(* Logix 5000 AddOnInstructionDefinition export AKD_Get_Parameter_LINT; software revision 19.01 *)

TYPE AKD_Status :   // All connections to the drive ethernet module are established and data is successfully transferring.
STRUCT
   Profile_In_Progress : BOOL;   // Profile Move In Progress
   Block_In_Execution : BOOL;   // Block In Execution
   On_Target_Position : BOOL;   // On Target Position (1=Current Position Equals Last Target Position)
   General_Fault : BOOL;   // General Fault
   Current_Direction : BOOL;   // Current Motor Direction (0=Reverse, 1=Forward)
   Home_Level : BOOL;   // Level of Home Input
   Reg_Level : BOOL;   // Level of Registration Input
   Enable : BOOL;   // State of Enable Output
   Fault_Input_Fault : BOOL;   // Fault Input Active
   Fwd_Limit : BOOL;   // Forward Input Active
   Rev_Limit : BOOL;   // Reverse Input Active
   Positive_Limit : BOOL;   // Positive Software Limit Exceeded
   Negative_Limit : BOOL;   // Negative Software Limit Exceeded
   FE_Fault : BOOL;   // Following Error Fault
   Block_Fault : BOOL;   // Block Execution Fault
   Load_Complete : BOOL;   // Command Message Successfully Loaded
END_STRUCT
END_TYPE

TYPE AKD_Control :   // Send Explicit Message
STRUCT
   Load_Data_Start_Profile : BOOL;   // Load Command Data / Start Profile Move
   Start_Block : BOOL;   // Execute Command block or block chain
   Incremental : BOOL;   // Incremental Position (0=Absolute, 1=Incremental)
   Direction : BOOL;   // Direction in Velocity Mode (0=Reverse, 1=Forward)
   Smooth_Stop : BOOL;   // Smooth / Controlled Stop w/ Deceleration
   Hard_Stop : BOOL;   // Hard / Immediate Stop
   Reg_Arm : BOOL;   // Arm the Registration Input
   Enable : BOOL;   // Enable Output
END_STRUCT
END_TYPE

TYPE AKD_Axis :   // Axis Data:
STRUCT
   Control : AKD_Control;   // Control bits to send to the drive
   Status : AKD_Status;   // Status bits received from the drive
   Input : AB:ETHERNET_MODULE_SINT_64Bytes:I:0;   // Data from the drive
   Output : AB:ETHERNET_MODULE_SINT_64Bytes:O:0;   // Data to the drive
   ResponseMsgType : SINT;   // Response type contained in latest IO response from drive. Used to check for errors
   CommandTimeout : INT;   // Time to allow for command response from drive. Dependent on scan rate and communicaiton rate
   PositionFeedback : DINT;   // Actual Position Value
   VelocityFeedback : DINT;   // Actual Velocity Value
END_STRUCT
END_TYPE

ADD_ON_INSTRUCTION AKD_Get_Parameter_LINT   (* revision 0.0, ExecutePrescan, ExecuteEnableInFalse *)
// Get 8 byte Drive Parameter
VAR_OUTPUT
   DN : BOOL; {access Read Only, visible}   // Command Successful
   ER : BOOL; {access Read Only, visible}   // Error
END_VAR
VAR_IN_OUT
   Axis : AKD_Axis; {required}
END_VAR
VAR_INPUT
   Parameter_Number : INT; {visible}   // See help (F1) for parameter list.
END_VAR
VAR_OUTPUT
   Parameter_Value_LSB : DINT; {access Read Only, required}   // Lower Parameter Value
   Parameter_Value_MSB : DINT; {access Read Only, required}   // Upper Parameter Value
END_VAR
VAR
   Command_Timeout : TIMER := (PRE := 2000);   // Timeout Timer
   Command_Message_Type : SINT;   // Command Message Type
   Command_Axis_Number : SINT;   // Command Axis Number
   Step : SINT;
   Command_Bytes : SINT[8];
   OS_LoadStart : BOOL;
   Temp_Bytes : SINT[2];   // Temporary Bytes to Split into Command Bytes
END_VAR

ROUTINE EnableInFalse   (* ladder *)
// EnableIn_False
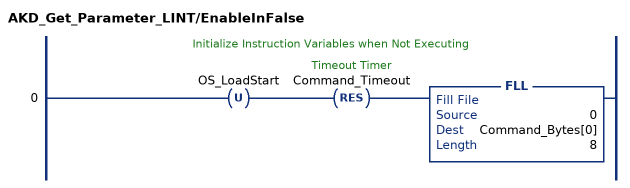
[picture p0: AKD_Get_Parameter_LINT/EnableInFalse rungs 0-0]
   // Initialize Instruction Variables when Not Executing
   0: OTU(OS_LoadStart)RES(Command_Timeout)FLL(0,Command_Bytes[0],8);
END_ROUTINE

ROUTINE Logic   (* ladder *)
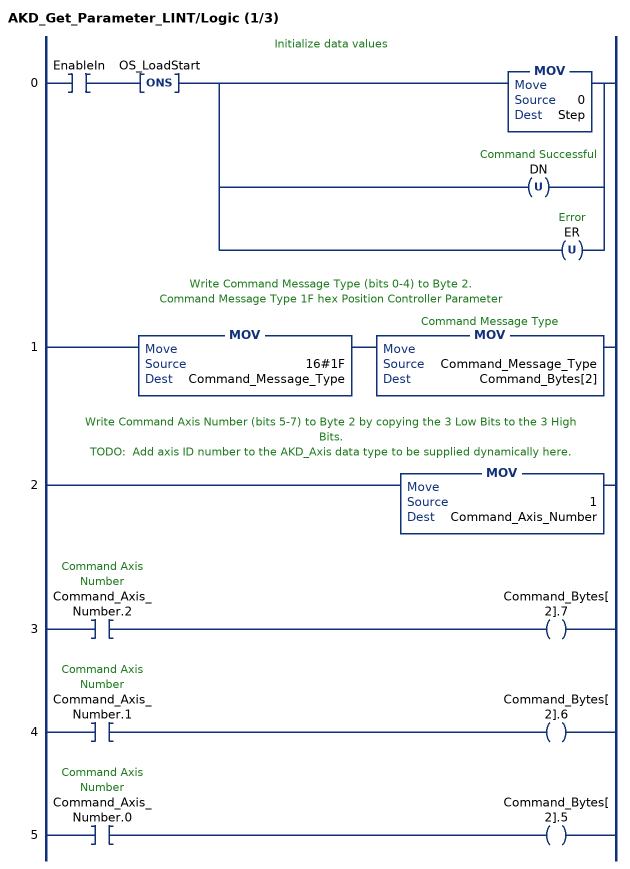
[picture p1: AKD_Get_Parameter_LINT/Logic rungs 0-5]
   // Initialize data values
   0: XIC(EnableIn)ONS(OS_LoadStart)[MOV(0,Step) ,OTU(DN) ,OTU(ER) ];
   // Write Command Message Type (bits 0-4) to Byte 2.
   // Command Message Type 1F hex Position Controller Parameter
   1: MOV(16#1F,Command_Message_Type)MOV(Command_Message_Type,Command_Bytes[2]);
   // Write Command Axis Number (bits 5-7) to Byte 2 by copying the 3 Low Bits to the 3 High Bits.
   // TODO:  Add axis ID number to the AKD_Axis data type to be supplied dynamically here.
   2: MOV(1,Command_Axis_Number);
   3: XIC(Command_Axis_Number.2)OTE(Command_Bytes[2].7);
   4: XIC(Command_Axis_Number.1)OTE(Command_Bytes[2].6);
   5: XIC(Command_Axis_Number.0)OTE(Command_Bytes[2].5);
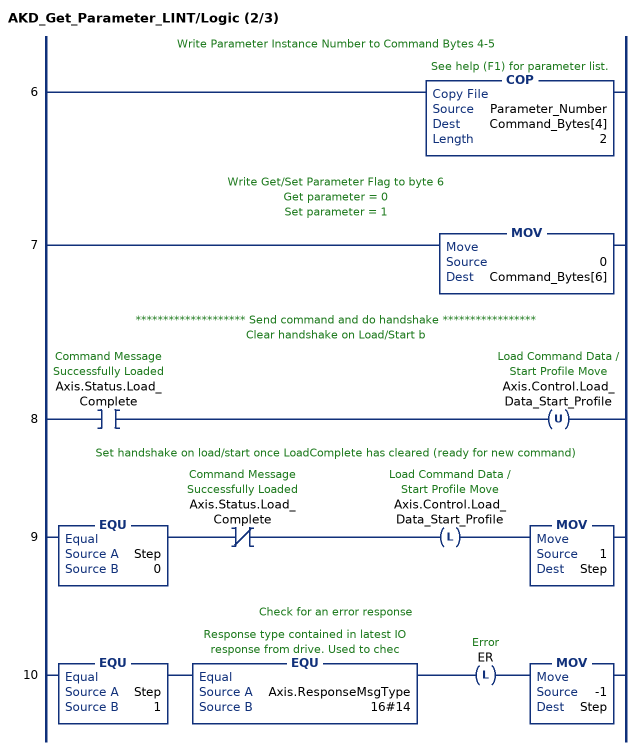
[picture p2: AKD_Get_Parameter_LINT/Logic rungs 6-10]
   // Write Parameter Instance Number to Command Bytes 4-5
   6: COP(Parameter_Number,Command_Bytes[4],2);
   // Write Get/Set Parameter Flag to byte 6
   // Get parameter = 0
   // Set parameter = 1
   7: MOV(0,Command_Bytes[6]);
   // ******************** Send command and do handshake *****************
   // Clear handshake on Load/Start b
   8: XIC(Axis.Status.Load_Complete)OTU(Axis.Control.Load_Data_Start_Profile);
   // Set handshake on load/start once LoadComplete has cleared (ready for new command)
   9: EQU(Step,0)XIO(Axis.Status.Load_Complete)OTL(Axis.Control.Load_Data_Start_Profile)MOV(1,Step);
   // Check for an error response
   10: EQU(Step,1)EQU(Axis.ResponseMsgType,16#14)OTL(ER)MOV(-1,Step);
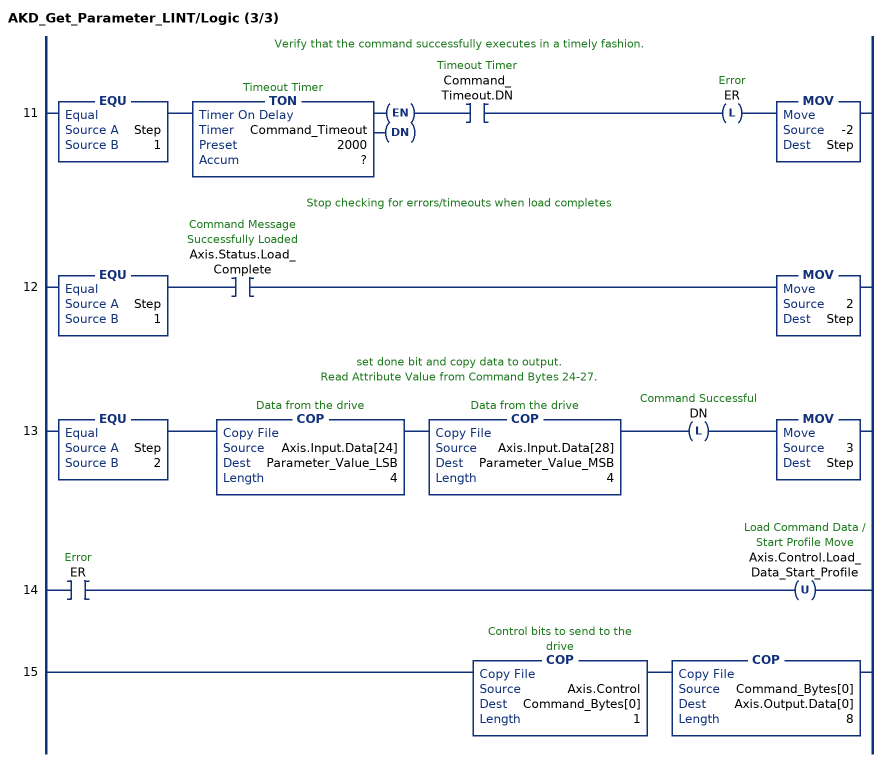
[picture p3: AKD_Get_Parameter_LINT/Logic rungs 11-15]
   // Verify that the command successfully executes in a timely fashion.
   11: EQU(Step,1)TON(Command_Timeout,?,?)XIC(Command_Timeout.DN)OTL(ER)MOV(-2,Step);
   // Stop checking for errors/timeouts when load completes
   12: EQU(Step,1)XIC(Axis.Status.Load_Complete)MOV(2,Step);
   // set done bit and copy data to output.
   // Read Attribute Value from Command Bytes 24-27.
   13: EQU(Step,2)COP(Axis.Input.Data[24],Parameter_Value_LSB,4)COP(Axis.Input.Data[28],Parameter_Value_MSB,4)OTL(DN)MOV(3,Step);
   14: XIC(ER)OTU(Axis.Control.Load_Data_Start_Profile);
   15: COP(Axis.Control,Command_Bytes[0],1)COP(Command_Bytes[0],Axis.Output.Data[0],8);
END_ROUTINE

ROUTINE Prescan   (* ladder *)
// Prescan
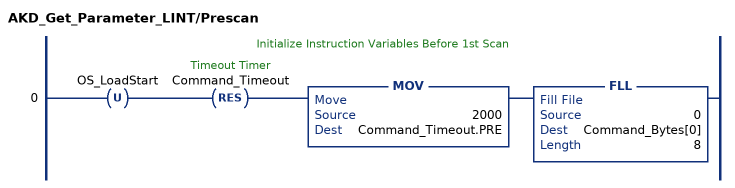
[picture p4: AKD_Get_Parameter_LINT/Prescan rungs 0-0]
   // Initialize Instruction Variables Before 1st Scan
   0: OTU(OS_LoadStart)RES(Command_Timeout)MOV(2000,Command_Timeout.PRE)FLL(0,Command_Bytes[0],8);
END_ROUTINE
END_ADD_ON_INSTRUCTION
